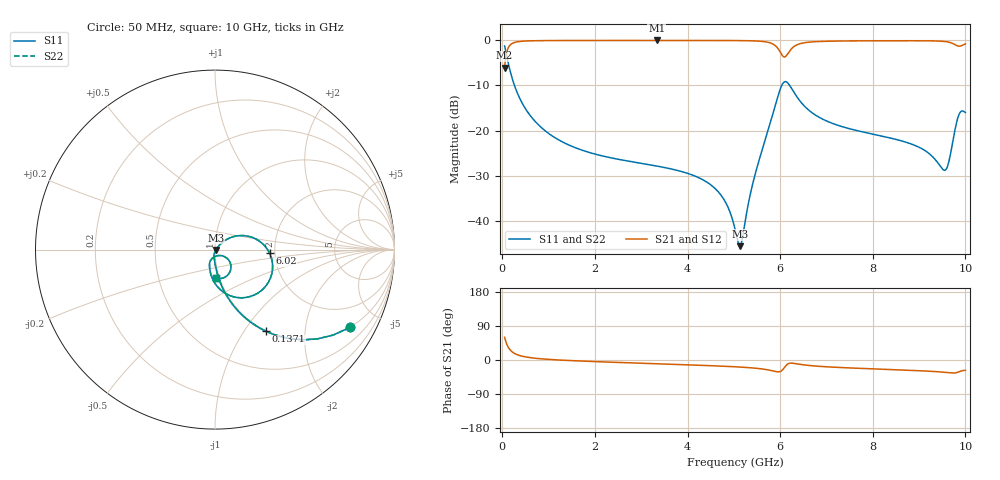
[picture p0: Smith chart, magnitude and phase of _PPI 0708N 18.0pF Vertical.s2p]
! S-Parameter data specifications (vertical orientation):
! Substrate: 40-mil Rogers 3003C, Substrate thickness, H=1.016mm, Dielectric constant, Er=3, Conductor thickness, T_mtl=0.043mm, Loss Tangent, Tand=0.003
! PCB Mounting Pad Footprint: Pad width, PadW=2.54mm , Pad length, PadL=0.51mm , Pad gap, PadG (edge-to-edge)=0.71mm , Reference planes=1.73mm apart
! Created Tue Jan 16 08:52:22 2018
# GHz S MA R 50
! 2 Port Network Data from SP1.SP block
! freq  magS11  angS11  magS21  angS21  magS12  angS12  magS22  angS22
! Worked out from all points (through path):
!   801 points, 50 MHz to 10 GHz, reference 50 ohm
!   highest |S21| = -0.01 dB at 3.333 GHz (marker M1); lowest = -6.1 dB at 50 MHz (marker M2)
!   group delay of S21, straight-line fit = 11.1 ps
!   lowest |S11| = -45.7 dB at 5.137 GHz (marker M3), VSWR 1.01, Z = 50.5 - j0.223 ohm
!   |S11| at or under -10 dB: 262.7 MHz to 6.034 GHz (5.771 GHz wide, 183 % of centre); 6.206 GHz to end of sweep
!   |S22| runs from -45.7 to -1.2 dB; largest |S21 - S12| = 0
!   S11 on the Smith chart (normalised r, x): 50 MHz: 0.99, -3.47; 137.1 MHz: 0.99, -1.27; 6.02 GHz: 1.87, -0.08; 10 GHz: 0.96, -0.31
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0.05  0.8674 -30.0  0.4975 60.0  0.4975 60.0  0.8674 -30.0
0.1370625  0.537 -58.0  0.8434 32.0  0.8434 32.0  0.537 -58.0
0.2863125  0.2927 -74.0  0.956 16.0  0.956 16.0  0.2927 -74.0
0.671875  0.1327 -84.8  0.9909 5.1  0.9909 5.1  0.1327 -84.8
1.716625  0.06068 -92.5  0.9977 -2.8  0.9977 -2.8  0.06068 -92.5
3.3335  0.04038 -99.0  0.9984 -9.9  0.9984 -9.9  0.04038 -99.0
3.370812  0.04005 -99.2  0.9984 -10.1  0.9984 -10.1  0.04005 -99.2
4.539937  0.02407 -101.0  0.9978 -15.2  0.9978 -15.2  0.02407 -101.0
4.826  0.01583 -96.7  0.9969 -16.7  0.9969 -16.7  0.01583 -96.7
5.025  0.008075 -78.0  0.9957 -17.9  0.9957 -17.9  0.008075 -78.0
5.136938  0.005211 -25.1  0.9946 -18.7  0.9946 -18.7  0.005211 -25.1
5.447875  0.03095 44.9  0.9869 -21.4  0.9869 -21.4  0.03095 44.9
5.87075  0.1726 26.9  0.894 -29.6  0.894 -29.6  0.1726 26.9
6.02  0.3048 -3.8  0.7161 -29.4  0.7161 -29.4  0.3048 -3.8
6.206563  0.3158 -57.8  0.7642 -8.6  0.7642 -8.6  0.3158 -57.8
6.691625  0.1572 -96.1  0.9627 -15.2  0.9627 -15.2  0.1572 -96.1
8.345812  0.08332 -111.3  0.9908 -25.0  0.9908 -25.0  0.08332 -111.3
9.067187  0.06254 -111.8  0.9903 -28.7  0.9903 -28.7  0.06254 -111.8
9.55225  0.03623 -74.5  0.9724 -32.4  0.9724 -32.4  0.03623 -74.5
9.639313  0.04432 -48.1  0.9567 -33.5  0.9567 -33.5  0.04432 -48.1
9.85075  0.1457 -54.0  0.8633 -31.6  0.8633 -31.6  0.1457 -54.0
10  0.1583 -88.9  0.9145 -27.3  0.9145 -27.3  0.1583 -88.9
